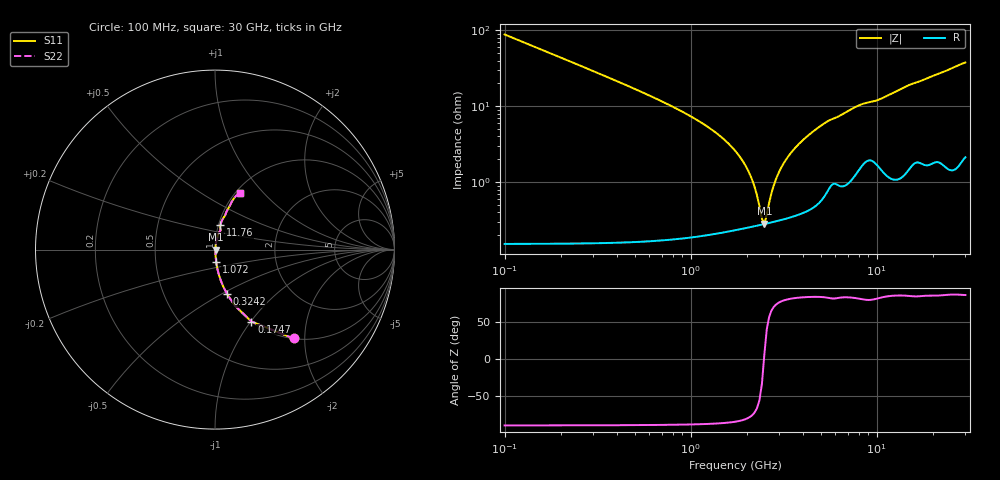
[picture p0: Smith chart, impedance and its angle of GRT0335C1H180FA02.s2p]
!Murata Part Number: GRT0335C1H180FA02
!These Parameters are Measured in Series Mode Connection
!Data Generated on Jun 19, 2026
!  o--ll--o
!Port1  Port2
!  o------o
!Operation Temp=25[degC], DC Bias Voltage=0[V]
!Freq. Start=100[MHz] Stop=30[GHz] 401[Steps]
# Hz S RI R 50
!Freq.(Hz) S11(Real) S11(Imag) S21(Real) S21(Imag) S12(Real) S12(Imag) S22(Real) S22(Imag)
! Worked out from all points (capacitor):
!   401 points, 100 MHz to 30 GHz, reference 50 ohm
!   read as one part in series: C = 18 pF near 249.5 MHz
!   lowest |Z| = 283 mohm at 2.492 GHz (marker M1)
!   series resonance near 2.48 GHz, so ESL is about 230 pH
!   S11 on the Smith chart (normalised r, x): 100 MHz: 1.00, -1.77; 174.8 MHz: 1.00, -1.01; 324.2 MHz: 1.00, -0.54; 1.072 GHz: 1.00, -0.13; 11.76 GHz: 1.02, +0.29; 30 GHz: 1.04, +0.75
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1e8  0.4381 -0.4953  0.5619 0.4953  0.5619 0.4953  0.4381 -0.4953
1.7475e8  0.2029 -0.4006  0.7971 0.4006  0.7971 0.4006  0.2029 -0.4006
3.2425e8  0.0682 -0.2492  0.9318 0.2492  0.9318 0.2492  0.0682 -0.2492
6.2325e8  0.0189 -0.13  0.9811 0.13  0.9811 0.13  0.0189 -0.13
1.07175e9  0.00633 -0.0663  0.9937 0.0663  0.9937 0.0663  0.00633 -0.0663
1.894e9  0.00279 -0.0192  0.9972 0.0192  0.9972 0.0192  0.00279 -0.0192
2.11825e9  0.00269 -0.0111  0.9973 0.0111  0.9973 0.0111  0.00269 -0.0111
2.3425e9  0.00272 -0.00402  0.9973 0.00402  0.9973 0.00402  0.00272 -0.00402
2.492e9  0.0028 0.000332  0.9972 -0.000332  0.9972 -0.000332  0.0028 0.000332
2.56675e9  0.00285 0.00241  0.9971 -0.00241  0.9971 -0.00241  0.00285 0.00241
2.791e9  0.00306 0.00832  0.9969 -0.00832  0.9969 -0.00832  0.00306 0.00832
2.9405e9  0.00323 0.012  0.9968 -0.012  0.9968 -0.012  0.00323 0.012
3.31425e9  0.00376 0.0207  0.9962 -0.0207  0.9962 -0.0207  0.00376 0.0207
4.06175e9  0.00527 0.0362  0.9947 -0.0362  0.9947 -0.0362  0.00527 0.0362
5.10825e9  0.00908 0.056  0.9909 -0.056  0.9909 -0.056  0.00908 0.056
7.7245e9  0.0215 0.0943  0.9785 -0.0943  0.9785 -0.0943  0.0215 0.0943
1.01165e10  0.0296 0.1141  0.9704 -0.1141  0.9704 -0.1141  0.0296 0.1141
1.1761e10  0.0305 0.1366  0.9695 -0.1366  0.9695 -0.1366  0.0305 0.1366
1.505e10  0.0486 0.1792  0.9514 -0.1792  0.9514 -0.1792  0.0486 0.1792
2.005825e10  0.0736 0.2281  0.9264 -0.2281  0.9264 -0.2281  0.0736 0.2281
2.50665e10  0.0996 0.2774  0.9004 -0.2774  0.9004 -0.2774  0.0996 0.2774
3e10  0.1382 0.3181  0.8618 -0.3181  0.8618 -0.3181  0.1382 0.3181
